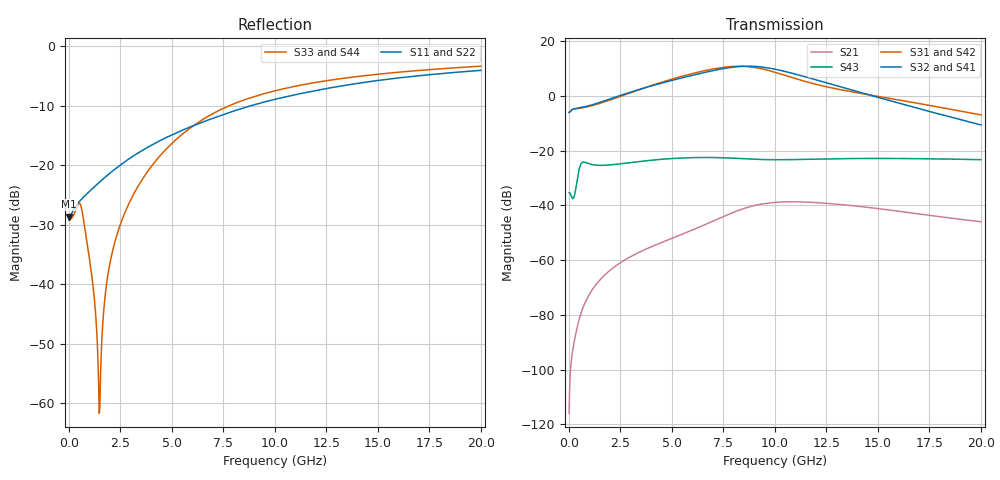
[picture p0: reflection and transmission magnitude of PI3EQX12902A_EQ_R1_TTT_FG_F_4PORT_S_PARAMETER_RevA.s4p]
! NPort=4 DATA=2000 NOISE=0 GROUPDELAY=0 COMPLEX_DATAFORMAT=POLAR
! NumOfBlock=1 NumOfParam=0
! .MODEL Smodel S TSTONEFILE=PI3EQX12902A_EQ_R1_TTT_FG_F_4PORT_S_PARAMETER_RevA.s4p TYPE=S
!  -- The above .MODEL line can be used for the S element in the netlist.
! The s parameter is extracted from the linear redriver, it is not bi-directional; only s(4,1)s(4,2) and s(3,1)s(3,2)
! should be the insertion loss
!Port definition:
!Port1 = input+
!Port2 = input-
!Port3 = output+
!Port4 = output-
# Hz S MA R  50
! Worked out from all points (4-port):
!   2000 points, 10 MHz to 20 GHz, reference 50 ohm
!   strongest paths, dB at 10 MHz, 5.01 GHz, 10.01 GHz, 15.01 GHz, 20 GHz:
!     S32: -6.0, 5.7, 9.7, -0.5, -10.6
!     S41: -6.0, 5.6, 9.6, -0.6, -10.6
!     S31: -6.0, 6.1, 8.6, -0.2, -7.0
!     S42: -6.0, 6.0, 8.4, -0.4, -7.0
!     S43: -35.3, -22.9, -23.3, -22.9, -23.3
!     S21: -116.0, -52.0, -38.9, -41.2, -46.0
!   lowest |S11| = -28.6 dB at 10 MHz (marker M1), VSWR 1.08, Z = 46.4 - j0.0607 ohm
!   |S11| at or under -10 dB: start of sweep to 8.837 GHz
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1e7  0.03704 -179.0  1.589e-06 51.9  0 0.0  0 0.0
     1.589e-06 51.9  0.03704 -179.0  0 0.0  0 0.0
     0.4994 1.0  0.4994 -179.0  0.03429 6.0  0.01709 -177.1
     0.4994 -179.0  0.4994 1.0  0.01709 -177.1  0.03429 6.0
5.88e9  0.2091 -112.1  0.003404 94.7  1.502e-06 -21.2  9.701e-07 88.8
        0.003402 94.6  0.2091 -112.1  9.708e-07 89.0  1.494e-06 -20.9
        2.496 -45.3  2.321 113.0  0.2045 -45.1  0.07385 146.0
        2.31 112.9  2.459 -45.9  0.07422 146.1  0.2039 -45.1
7.67e9  0.2727 -111.7  0.006684 78.3  5.58e-06 -75.0  3.682e-06 44.4
        0.006665 78.3  0.2726 -111.7  3.68e-06 44.5  5.552e-06 -74.5
        3.379 -95.8  3.228 61.1  0.3101 -63.1  0.07311 126.9
        3.203 61.0  3.315 -96.2  0.07359 126.9  0.3094 -63.0
9.16e9  0.328 -113.2  0.01029 48.6  1.079e-05 -122.6  8.531e-06 -7.1
        0.01025 48.7  0.328 -113.1  8.499e-06 -7.1  1.076e-05 -121.9
        3.238 -146.5  3.43 6.6  0.385 -75.4  0.06883 115.4
        3.392 6.7  3.165 -146.8  0.06927 115.2  0.3846 -75.3
1.086e10  0.3868 -115.7  0.01165 12.1  1.586e-05 -164.0  1.384e-05 -66.8
          0.01161 12.3  0.3868 -115.7  1.374e-05 -66.7  1.592e-05 -163.1
          2.149 168.2  2.575 -50.8  0.4562 -86.6  0.06827 106.2
          2.543 -50.4  2.093 168.2  0.06853 105.9  0.4563 -86.5
1.341e10  0.4686 -120.0  0.01018 -27.4  2.534e-05 149.8  1.825e-05 -137.3
          0.01018 -27.0  0.4687 -120.0  1.803e-05 -136.9  2.563e-05 150.5
          1.25 128.8  1.388 -114.4  0.5398 -99.4  0.0714 89.4
          1.375 -113.6  1.22 129.4  0.07138 89.1  0.5402 -99.3
2e10  0.6265 -131.6  0.004946 -73.3  4.228e-05 50.4  1.767e-05 101.1
      0.005025 -73.3  0.6265 -131.6  1.739e-05 102.4  4.291e-05 50.5
      0.4491 40.6  0.2947 134.4  0.6794 -119.6  0.06844 46.2
      0.2954 135.4  0.4445 41.5  0.06835 46.1  0.6797 -119.6
